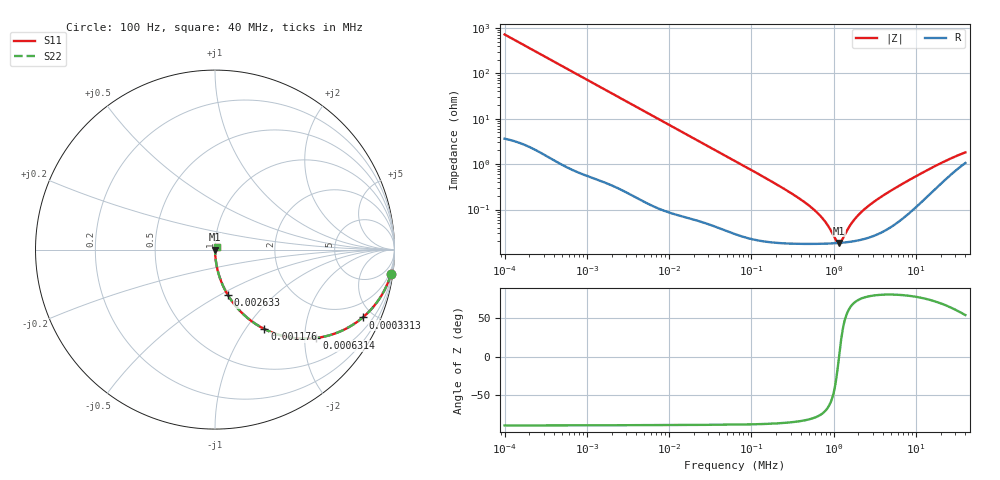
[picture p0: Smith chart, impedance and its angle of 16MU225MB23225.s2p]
!Components F PML CAP
!CONCATENATE F 0.1-40000kHz, at 20deg DC=0V
!Part Number F 16MU225MB23225
!Copyright(C) Rubycon Corporation. 20161128
# MHz S MA R 50
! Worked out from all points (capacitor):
!   561 points, 100 Hz to 40 MHz, reference 50 ohm
!   read as one part in series: C = 2.22 uF near 104.7 Hz
!   lowest |Z| = 18.4 mohm at 1.152 MHz (marker M1)
!   series resonance near 1.164 MHz, so ESL is about 8.4 nH
!   S11 on the Smith chart (normalised r, x): 100 Hz: 1, -14; 331.3 Hz: 1.03, -4.34; 631.4 Hz: 1.02, -2.28; 1.176 kHz: 1.01, -1.23; 2.633 kHz: 1.01, -0.55; 40 MHz: 1.02, +0.03
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0.0001  0.9897 -8.0  0.1385 81.7  0.1385 81.7  0.9897 -8.0
0.0001950324  0.9633 -15.2  0.262 74.4  0.262 74.4  0.9633 -15.2
0.000331277  0.9059 -24.7  0.4174 64.9  0.4174 64.9  0.9059 -24.7
0.000631385  0.7496 -41.1  0.6567 48.6  0.6567 48.6  0.7496 -41.1
0.0008716573  0.6353 -50.1  0.7676 39.4  0.7676 39.4  0.6353 -50.1
0.001175963  0.5216 -58.1  0.849 31.4  0.849 31.4  0.5216 -58.1
0.001739627  0.383 -67.0  0.9203 22.5  0.9203 22.5  0.383 -67.0
0.002633433  0.2651 -74.1  0.9616 15.4  0.9616 15.4  0.2651 -74.1
0.007424854  0.09777 -83.8  0.9942 5.6  0.9942 5.6  0.09777 -83.8
0.06324555  0.01172 -87.9  0.9996 0.7  0.9996 0.7  0.01172 -87.9
0.2699366  0.002624 -85.9  0.9998 0.1  0.9998 0.1  0.002624 -85.9
0.5512845  0.001065 -80.5  0.9998 0.1  0.9998 0.1  0.001065 -80.5
0.778809  0.0005585 -71.5  0.9998 0.0  0.9998 0.0  0.0005585 -71.5
1.075183  0.0002085 -29.3  0.9998 0.0  0.9998 0.0  0.0002085 -29.3
1.152109  0.0001839 -4.1  0.9998 0.0  0.9998 0.0  0.0001839 -4.1
1.234538  0.0002 22.2  0.9998 -0.0  0.9998 -0.0  0.0002 22.2
1.590541  0.0004512 64.4  0.9998 -0.0  0.9998 -0.0  0.0004512 64.4
2.049205  0.0007928 74.5  0.9998 -0.0  0.9998 -0.0  0.0007928 74.5
2.894947  0.001358 79.2  0.9997 -0.1  0.9997 -0.1  0.001358 79.2
4.69589  0.002443 80.8  0.9996 -0.1  0.9996 -0.1  0.002443 80.8
16.66941  0.008802 71.9  0.9973 -0.5  0.9973 -0.5  0.008802 71.9
40  0.01789 53.3  0.9894 -0.8  0.9894 -0.8  0.01789 53.3
